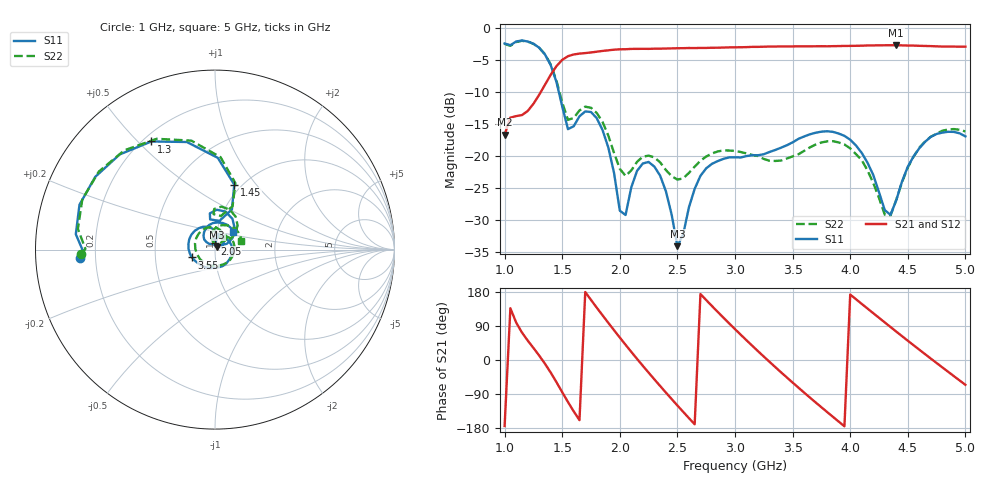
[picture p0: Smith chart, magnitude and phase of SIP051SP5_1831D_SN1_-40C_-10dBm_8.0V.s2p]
# GHz  S  dB  R  50
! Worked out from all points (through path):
!   81 points, 1 GHz to 5 GHz, reference 50 ohm
!   highest |S21| = -2.73 dB at 4.4 GHz (marker M1); lowest = -16.7 dB at 1 GHz (marker M2)
!   lowest |S11| = -34.1 dB at 2.5 GHz (marker M3), VSWR 1.04, Z = 51.3 + j1.56 ohm
!   |S11| at or under -10 dB: 1.47 GHz to end of sweep
!   |S22| runs from -29.3 to -2.0 dB; largest |S21 - S12| = 0.0026
!   S11 on the Smith chart (normalised r, x): 1 GHz: 0.14, -0.03; 1.3 GHz: 0.23, +0.55; 1.45 GHz: 0.92, +0.78; 2.05 GHz: 1.00, +0.07; 3.55 GHz: 0.77, -0.07; 5 GHz: 1.20, +0.24
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1  -2.46 -176.4  -16.70 -174.4  -16.73 -174.2  -2.52 -178.1
1.15  -1.99 161.7  -13.63 72.8  -13.63 72.9  -2.04 159.3
1.3  -3.11 120.4  -10.47 11.7  -10.45 11.7  -3.13 117.7
1.45  -8.45 73.5  -6.01 -58.5  -5.99 -58.5  -8.24 72.9
1.55  -15.82 81.1  -4.45 -110.9  -4.44 -110.9  -14.38 79.7
1.7  -13.06 87.5  -3.96 179.5  -3.94 179.5  -12.31 81.4
1.9  -18.67 33.2  -3.53 98.2  -3.50 98.3  -16.81 38.1
2.05  -29.21 91.4  -3.36 40.1  -3.35 40.1  -23.12 57.6
2.2  -21.18 82.0  -3.29 -15.4  -3.30 -15.3  -20.12 63.0
2.35  -23.08 43.0  -3.27 -68.5  -3.26 -68.5  -21.00 44.9
2.5  -34.08 50.5  -3.20 -120.0  -3.20 -120.0  -23.69 48.4
2.7  -23.10 80.4  -3.16 174.1  -3.15 174.1  -20.75 52.1
2.85  -20.80 32.8  -3.12 126.9  -3.11 126.9  -19.30 31.0
3  -20.22 -16.9  -3.06 81.4  -3.05 81.4  -19.23 3.1
3.25  -19.73 -93.8  -2.96 9.0  -2.95 9.1  -20.47 -60.0
3.55  -17.34 -161.2  -2.90 -72.8  -2.90 -72.8  -19.75 -164.7
3.7  -16.39 167.8  -2.90 -111.9  -2.90 -111.9  -18.23 148.6
4  -17.47 108.2  -2.84 172.7  -2.83 172.7  -18.82 77.3
4.35  -29.20 116.3  -2.74 87.1  -2.75 87.1  -29.29 89.1
4.4  -26.90 134.8  -2.73 75.0  -2.74 75.0  -26.85 103.9
4.7  -17.02 103.6  -2.87 3.7  -2.86 3.8  -17.01 74.6
5  -16.95 44.1  -2.96 -65.5  -2.96 -65.6  -16.18 18.9
